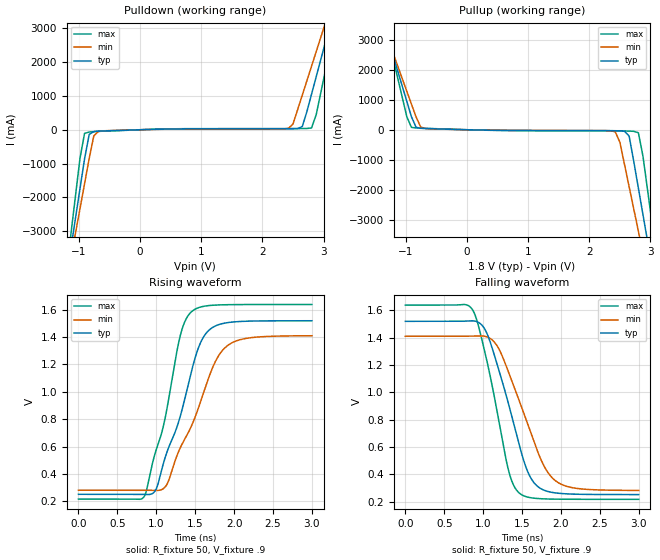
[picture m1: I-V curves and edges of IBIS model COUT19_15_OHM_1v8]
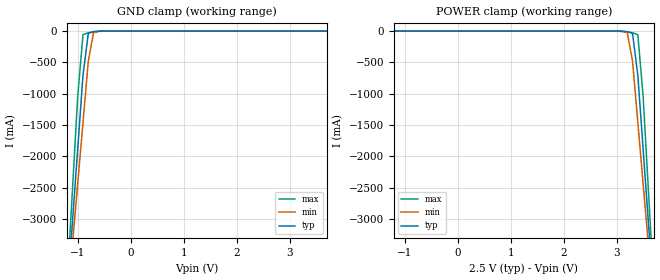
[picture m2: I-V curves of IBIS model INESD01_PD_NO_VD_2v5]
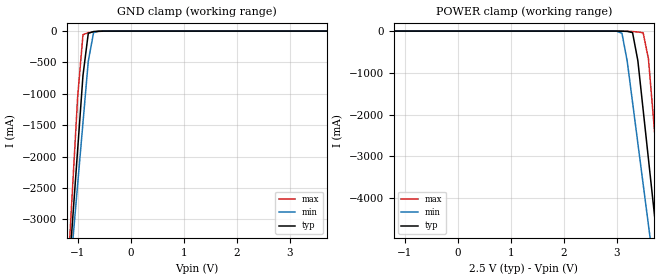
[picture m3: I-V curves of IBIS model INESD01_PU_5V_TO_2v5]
|   This file is an IBIS representation of the   |
|   Integrated Device Technology , Inc.   |
|   ICS83052i   |
|   2:1, SINGLE-ENDED MULTIPLEXER   |
[IBIS Ver]   4.1
[File name]   83052i.ibs
[File Rev]   1.0
[Date]   15 Mar 2010
[Source]   Originated at Integrated Device Technology, Inc.
[Disclaimer]
IDT hereby grants the user of this IBIS model a non-exclusive,
nontransferable license to use this IBIS model under the following terms.
Before using this IBIS model, the user should read this license.
If the user does not accept these terms,  the IBIS model should be
returned to IDT within 30 days.
   The user is granted this license only to use the IBIS model and
is not granted rights to sell, load, rent, lease or license the IBIS
model in whole or in part, or in modified form to anyone other than
user. User may modify the IBIS model to suit its specific
applications but rights to derivative works and such modifications
shall belong to IDT.
   This IBIS model is provided on an "AS IS" basis and IDT makes
absolutely no warranty with respect to the information contained
herein. IDT DISCLAIMS AND CUSTOMER WAIVES ALL WARRANTIES, EXPRESS
OR IMPLIED, INCLUDING WARRANTIES OF MERCHANTABILITY OR FITNESS FOR
A PARTICULAR PURPOSE. The entire risk as to quality and performance
is with the Customer. ACCORDINGLY, IN NO EVENT SHALL THE COMPANY BE
LIABLE FOR ANY DAMAGES, WHETHER IN CONTRACT OR TORT,INCLUDING ANY
LOST PROFITS OR OTHER INCIDENTAL, CONSEQUENTIAL, EXEMPLARY, OR
PUNITIVE DAMAGES ARISING OUT OF THE USE OR APPLICATION OF THE IBIS
model provided in this package. Further, IDT reserves the right to
make changes without notice to any product herein to improve
reliability, function, or design. IDT does not convey any license
under patent rights or any other intellectual property rights,
including those of third parties.
   IDT is not obligated to provide maintenance or support
for the licensed IBIS model.
[Copyright]   Copyright 2006 by Integrated Device Technology, Inc.
[Component]   ICS83052AGI
[Manufacturer] Integrated Device Technology, Inc.
[Package]
|TSSOP 8 Lead
|   typ   min   max
R_pkg   52.5m   48.8m   56.2m
L_pkg   1.381nH   1.275nH   1.486nH
C_pkg   0.236pF   0.230pF   0.242pF
[Pin] signal_name  model_name   R_pin   L_pin   C_pin
1   VDDO   POWER   56.2m   1.486n   0.242p
2   GND   GND   48.8m   1.275n   0.230p
3   CLK1   INESD01_PD_NO_VD   48.8m   1.275n   0.230p
4   VDD   POWER   56.2m   1.468n   0.242p
5   OE   INESD01_PU_5V_TO   56.2m   1.486n   0.242p
6   CLK0   INESD01_PD_NO_VD   48.8m   1.275n   0.230p
7   SEL0   INESD01_PD_5V_TO   48.8m   1.275n   0.230p
8   Q   COUT19_15_OHM   56.2m   1.468n   0.242p
[Model Selector] INESD01_PD_NO_VD
INESD01_PD_NO_VD_2v5  Buffer selection for 2v5
INESD01_PD_NO_VD_3v3  Buffer selection for 3v3
[Model Selector] INESD01_PU_5V_TO
INESD01_PU_5V_TO_2v5  Buffer selection for 2v5
INESD01_PU_5V_TO_3v3  Buffer selection for 3v3
[Model Selector] INESD01_PD_5V_TO
INESD01_PD_5V_TO_2v5  Buffer selection for 2v5
INESD01_PD_5V_TO_3v3  Buffer selection for 3v3
[Model Selector] COUT19_15_OHM
COUT19_15_OHM_1v8  Buffer selection for 1v8
COUT19_15_OHM_2v5  Buffer selection for 2v5
COUT19_15_OHM_3v3  Buffer selection for 3v3
| Models and submodels in the file (9): COUT19_15_OHM_1v8 (Output), INESD01_PD_NO_VD_2v5 (Input), INESD01_PU_5V_TO_2v5 (Input), INESD01_PD_5V_TO_2v5 (Input), COUT19_15_OHM_2v5 (Output), INESD01_PD_NO_VD_3v3 (Input), INESD01_PU_5V_TO_3v3 (Input), INESD01_PD_5V_TO_3v3 (Input), COUT19_15_OHM_3v3 (Output)
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[Model] COUT19_15_OHM_1v8
Model_type   Output
Polarity   Non-Inverting
|   typ   min   max
C_comp   2pF   1.5pF   2.5pF
Vmeas = .9
Rref = 50
Cref = 0
Vref = .9
|   typ   min   max
[Voltage range]   1.8V   1.710V   1.890V
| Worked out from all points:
|   slope of the pulldown table from 0 to 0.27 V, typ, clamps not added: 19.8 ohm
|   slope of the pullup table from 0 to 0.27 V, typ, clamps not added: 22.6 ohm
|   rising waveform, R_fixture 50, V_fixture .9: 20-80 % time 403ps typ, 481ps min, 324ps max; typ from 0.252 V to 1.52 V
|   falling waveform, R_fixture 50, V_fixture .9: 20-80 % time 371ps typ, 441ps min, 300ps max; typ from 1.52 V to 0.252 V
[Pulldown]
|Voltage   I (typ)   I (min)   I (max)
-2.5V     -19.66A    -17.26A    -23.71A
-1.136V   -3.543A    -3.832A    -3.14A
-1.061V   -2.648A    -3.086A    -1.997A
-909.1mV  -857.9mA   -1.595A    -108.7mA
-833.3mV  -138.7mA   -849.6mA   -66.84mA
-681.8mV  -42.67mA   -49.14mA   -48.79mA
2.424V    28.84mA    38.68mA    34.53mA
2.652V    93.41mA    1.019A     35.21mA
2.803V    1.047A     1.874A     53.51mA
3.03V     2.585A     3.158A     1.747A
3.182V    3.613A     4.015A     3.059A
5V        16A        14.34A     18.86A
[Pullup]
|Voltage   I (typ)   I (min)   I (max)
-2.5V     11.27A     9.895A     13.61A
-1.364V   3.527A     3.434A     3.725A
-909.1mV  434.4mA    855.6mA    78.42mA
-681.8mV  40.75mA    40.24mA    47.98mA
2.424V    -33.24mA   -67.99mA   -35.9mA
2.5V      -37.47mA   -416mA     -37.07mA
2.652V    -212.3mA   -1.903A    -45.59mA
2.803V    -1.953A    -3.392A    -100.3mA
2.955V    -3.741A    -4.882A    -2.038A
3.03V     -4.635A    -5.627A    -3.18A
3.106V    -5.529A    -6.373A    -4.322A
5V        -27.9A     -25.02A    -32.88A
[Ramp]
|   typ   min   max
dV/dt_r   1.014/0.553n   0.903/0.658n   1.137/0.45n
dV/dt_f   1.016/0.533n   0.904/0.637n   1.139/0.429n
R_load =   50.0000
[Rising Waveform]
R_fixture = 50
V_fixture = .9   |Vcc_typ
V_fixture_min = .855 |Vcc_min
V_fixture_max = .945 |Vcc_max
C_fixture = 0.0p
| Time   typ   min   max
0s        252.4mV    282.3mV    217.7mV
846.8ps   251.5mV    282.5mV    238.5mV
1.009ns   305.2mV    280.3mV    594.7mV
1.138ns   562mV      326.2mV    879.1mV
1.312ns   829.5mV    596.8mV    1.419V
1.459ns   1.165V     760.3mV    1.588V
1.637ns   1.425V     1.043V     1.627V
1.775ns   1.485V     1.238V     1.634V
1.919ns   1.506V     1.339V     1.636V
3ns       1.519V     1.41V      1.638V
[Falling Waveform]
R_fixture = 50
V_fixture = .9   |Vcc_typ
V_fixture_min = .855 |Vcc_min
V_fixture_max = .945 |Vcc_max
C_fixture = 0.0p
| Time   typ   min   max
0s        1.519V     1.41V      1.638V
867.9ps   1.523V     1.411V     1.599V
1.072ns   1.398V     1.4V       1.169V
1.192ns   1.181V     1.328V     821.1mV
1.321ns   925.8mV    1.155V     440.6mV
1.465ns   612.2mV    936.3mV    263.3mV
1.649ns   342.8mV    646mV      226.5mV
1.793ns   282.2mV    450.6mV    220.8mV
1.934ns   264.3mV    351.7mV    218.9mV
3ns       252.5mV    282.8mV    217.7mV
[Model] INESD01_PD_NO_VD_2v5
Model_type   Input
Polarity   Non-Inverting
Vinl = 0.80V
Vinh = 2.0V
|   typ   min   max
C_comp   2pF   1.5pF   2.5pF
|   typ   min   max
[Voltage range]  2.5V   2.375V   2.625V
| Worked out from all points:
|   GND clamp passes 1 mA (typ) near -0.53 V on its own axis
[GND_clamp]
|Voltage I(typ)   I(min)   I(max)
-2.5V     -19.61A    -17.19A    -23.68A
-1.2V     -4.247A    -4.404A    -4.063A
-1.1V     -3.067A    -3.422A    -2.554A
-1V       -1.887A    -2.441A    -1.045A
-900mV    -707.9mA   -1.461A    -58.38mA
-800mV    -36.14mA   -481.4mA   -25.07mA
-700mV    -7.313mA   -24.33mA   -13.7mA
-600mV    -2.207mA   -1.763mA   -5.095mA
-500mV    -388.3uA   -196.9uA   -934.5uA
5V        97.41uA    121.8uA    92.26uA
[POWER_clamp]
|Voltage   I(typ)   I(min)   I(max)
-2.5V     97.41uA    121.8uA    92.26uA
3V        -388.3uA   -196.9uA   -934.5uA
3.1V      -2.207mA   -1.763mA   -5.095mA
3.2V      -7.314mA   -24.33mA   -13.7mA
3.3V      -36.14mA   -481.4mA   -25.07mA
3.4V      -707.9mA   -1.461A    -58.38mA
3.5V      -1.887A    -2.441A    -1.045A
3.6V      -3.067A    -3.422A    -2.554A
3.7V      -4.247A    -4.404A    -4.063A
5V        -19.61A    -17.19A    -23.68A
[Model] INESD01_PU_5V_TO_2v5
Model_type   Input
Polarity   Non-Inverting
Vinl = 1.4V
Vinh = 1.85V
|   typ   min   max
C_comp   2pF   1.5pF   2.5pF
|   typ   min   max
[Voltage range]  2.5V   2.375V   2.625V
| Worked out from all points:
|   GND clamp passes 1 mA (typ) near -0.54 V on its own axis
[GND_clamp]
|Voltage   I(typ)   I(min)   I(max)
-2.5V     -19.6A     -17.18A    -23.67A
-1.2V     -4.246A    -4.402A    -4.061A
-1.1V     -3.066A    -3.421A    -2.553A
-1V       -1.886A    -2.44A     -1.044A
-900mV    -707.1mA   -1.46A     -57.44mA
-800mV    -35.62mA   -480.7mA   -24.4mA
-700mV    -7.027mA   -24.05mA   -13.29mA
-600mV    -2.107mA   -1.716mA   -4.908mA
-500mV    -400.3uA   -236.5uA   -910.3uA
5V        48.71uA    63.95uA    43.82uA
[POWER_clamp]
|Voltage   I(typ)   I(min)   I(max)
-2.5V     48.71uA    60.9uA     46.13uA
2.9V      -89.46uA   -362.8uA   -54.59uA
3.1V      -2.107mA   -51.03mA   -544.9uA
3.2V      -7.027mA   -725.4mA   -3.459mA
3.3V      -35.62mA   -1.705A    -10.87mA
3.4V      -707.1mA   -2.685A    -21.4mA
3.5V      -1.886A    -3.666A    -39.42mA
3.6V      -3.066A    -4.647A    -666.9mA
3.7V      -4.246A    -5.63A     -2.175A
3.8V      -5.426A    -6.612A    -3.684A
3.9V      -6.607A    -7.595A    -5.193A
5V        -19.6A     -18.41A    -21.79A
